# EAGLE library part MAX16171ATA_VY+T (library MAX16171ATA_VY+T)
Ideal Diode Controller with Reverse-Current Protection, 8 TDFN-CU Source: Datasheet
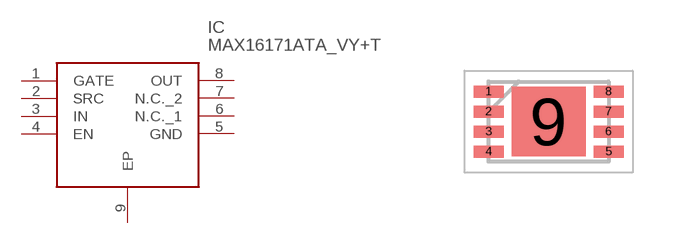
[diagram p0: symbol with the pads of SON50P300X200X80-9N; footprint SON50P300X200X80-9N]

Designator prefix IC

## MAX16171ATA_VY+T (Description: Ideal Diode Controller with Reverse-Current Protection, 8 TDFN-CU; Height: 0.8mm; Manufacturer_Name: Analog Devices; Manufacturer_Part_Number: MAX16171ATA/VY+T; Mouser_Part_Number: 700-MAX16171ATA/VY+T; Mouser_Price-Stock: https://www.mouser.co.uk/ProductDetail/Maxim-Integrated/MAX16171ATA-VY%2bT?qs=zW32dvEIR3uJUsRKfY9NHQ%3D%3D)  [SON50P300X200X80-9N]
1  GATE
2  SRC
3  IN
4  EN
5  GND
6  N.C._1
7  N.C._2
8  OUT
9  EP

## Footprint SON50P300X200X80-9N (pad centres in mm)
T823Y+3C
smd 0.75 x 0.3: 1 -1.5,0.75; 2 -1.5,0.25; 3 -1.5,-0.25; 4 -1.5,-0.75; 5 1.5,-0.75; 6 1.5,-0.25; 7 1.5,0.25; 8 1.5,0.75
smd 1.85 x 1.73: 9 0,0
